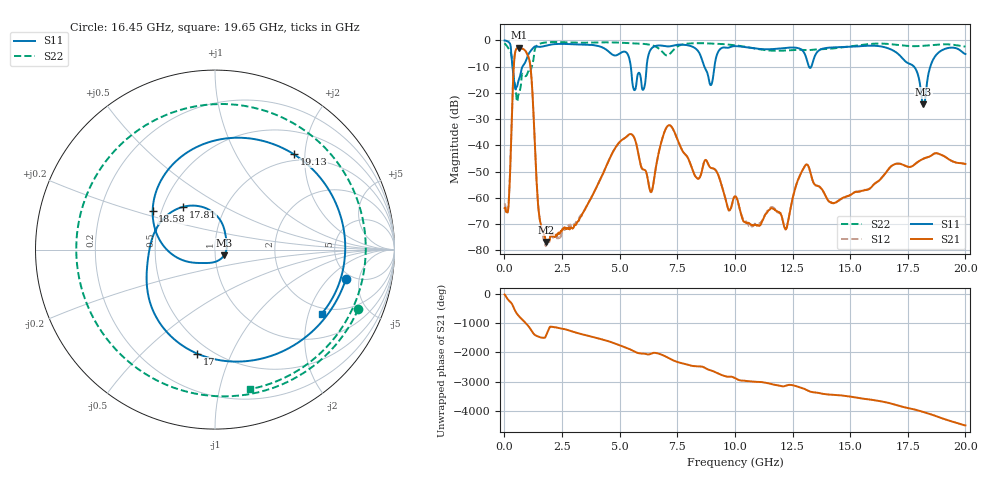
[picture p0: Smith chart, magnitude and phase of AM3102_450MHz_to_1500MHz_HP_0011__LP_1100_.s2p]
!Agilent Technologies,E8364B,MY43040894,A.07.50.67
!Agilent E8364B: A.07.50.67
!Date: Thursday, January 11, 2018 05:33:22
!Correction: S11(Full 2 Port(1,2))
!S21(Full 2 Port(1,2))
!S12(Full 2 Port(1,2))
!S22(Full 2 Port(1,2))
!S2P File: Measurements: S11, S21, S12, S22:
# Hz S  dB  R 50
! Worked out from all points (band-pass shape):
!   1601 points, 10 MHz to 20 GHz, reference 50 ohm
!   highest |S21| = -2.85 dB at 634.7 MHz (marker M1); lowest = -76.8 dB at 1.809 GHz (marker M2)
!   |S21| within 3 dB of the highest: 446.4 MHz to 1.02 GHz (573.6 MHz wide, 78.2 % of centre)
!   lowest |S11| = -24.4 dB at 18.18 GHz (marker M3), VSWR 1.13, Z = 55.3 - j3.49 ohm
!   |S11| at or under -10 dB: 353.4 MHz to 786.8 MHz (433.4 MHz wide, 76 % of centre); 5.485 GHz to 6.169 GHz (684.4 MHz wide, 11.7 % of centre); 17.77 GHz to 18.48 GHz (710.5 MHz wide, 3.92 % of centre)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
!   |S22| runs from -23.3 to -0.6 dB; largest |S21 - S12| = 0.0031
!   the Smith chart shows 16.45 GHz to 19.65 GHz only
!   S11 on the Smith chart (normalised r, x): 16.45 GHz: 4.41, -3.27; 17 GHz: 0.42, -0.75; 17.81 GHz: 0.63, +0.33; 18.58 GHz: 0.45, +0.23; 19.13 GHz: 0.88, +1.78; 19.65 GHz: 1.77, -2.44
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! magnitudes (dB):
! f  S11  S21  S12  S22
! 10 MHz  -0.1  -63.9  -62.1  -1.1
! 634.7 MHz  -14.8  -2.9  -2.9  -20.1
! 1.109 GHz  -4.4  -8.7  -8.7  -12.1
! 1.484 GHz  -2.5  -64.8  -64.4  -1.5
! 1.809 GHz  -2.0  -76.8  -77.9  -0.8
! 3.346 GHz  -1.6  -66.9  -66.5  -0.9
! 5.095 GHz  -4.5  -38.0  -38.0  -0.9
! 6.032 GHz  -18.8  -49.2  -49.3  -1.3
! 6.682 GHz  -2.0  -43.4  -43.4  -3.0
! 8.956 GHz  -17.1  -48.6  -48.6  -1.2
! 10.01 GHz  -2.2  -59.5  -59.5  -1.9
! 12.2 GHz  -2.9  -71.9  -71.6  -3.9
! 13.34 GHz  -9.5  -52.5  -52.6  -3.6
! 16.45 GHz  -2.5  -51.5  -51.5  -1.3
! 16.68 GHz  -3.1  -48.9  -48.9  -1.4
! 17 GHz  -4.6  -47.0  -47.0  -1.7
! 17.81 GHz  -10.5  -47.2  -47.1  -2.2
! 18.18 GHz  -24.4  -45.1  -45.1  -2.1
! 18.58 GHz  -7.8  -43.5  -43.6  -1.8
! 19.13 GHz  -3.2  -44.4  -44.4  -1.5
! 19.65 GHz  -3.2  -46.7  -46.7  -1.9
! 20 GHz  -5.2  -47.1  -47.2  -2.4
